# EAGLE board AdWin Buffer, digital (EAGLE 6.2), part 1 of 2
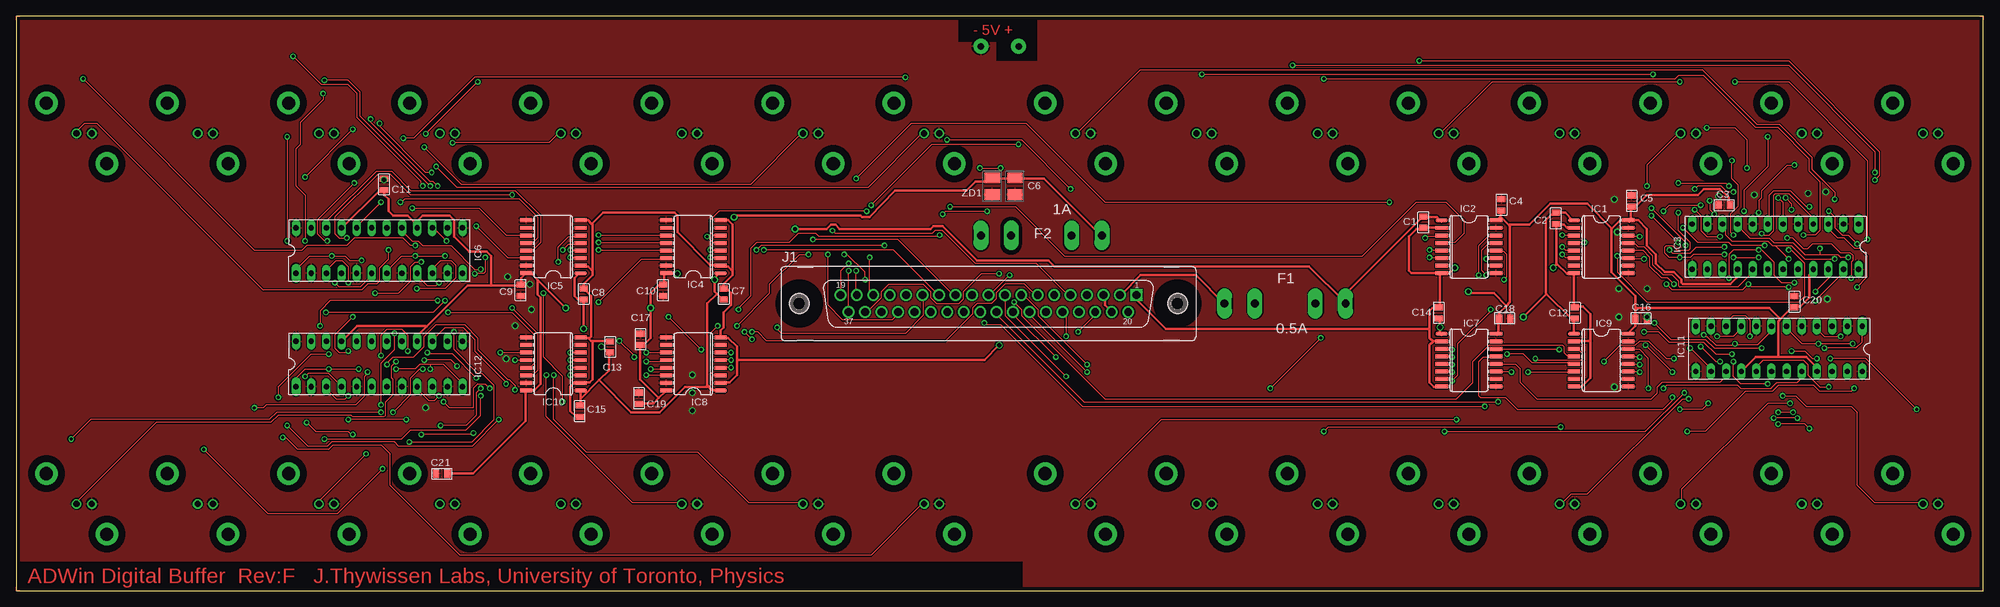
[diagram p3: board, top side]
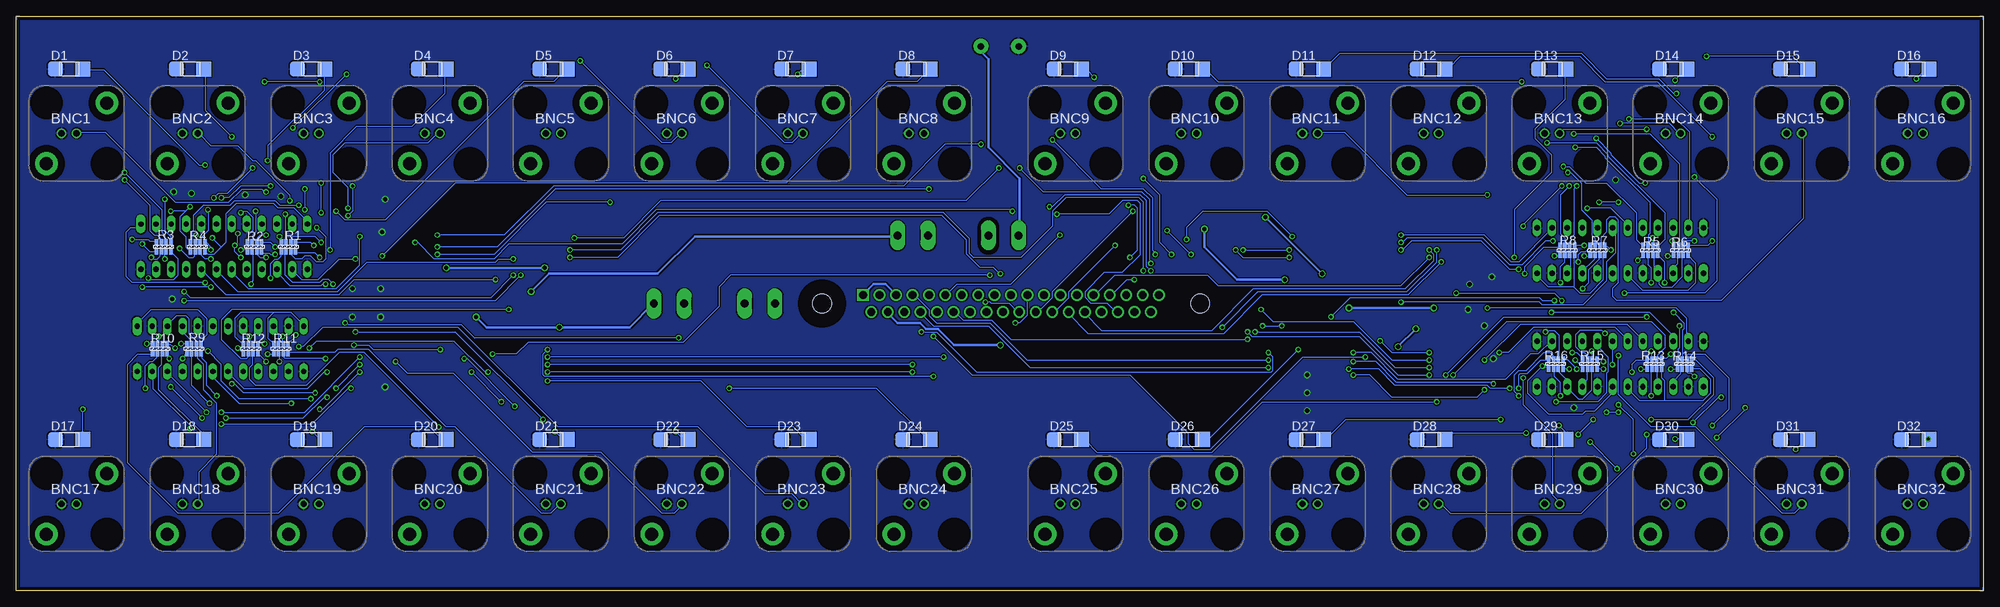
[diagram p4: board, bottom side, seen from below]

Size 330.2 x 96.52 mm. Coordinates in mm from the lower left corner, seen from the top.
Outline: 0,0 330.2,0 330.2,96.52 0,96.52 0,0
Copper layers (1+16): Top 0.035mm / dielectric 1.5mm / Bottom 0.035mm
Design rules: minimum track width 7mil, minimum drill 20mil, track to track 7mil, track to pad 7mil, pad to pad 7mil, via to via 7mil, smd to smd 0mil, copper to edge 25mil, drill to drill 8mil, minimum pad ring 10mil, minimum via ring 8mil, stop-mask expansion 4mil, vias tented up to drill 0mil, thermal gap 10mil
Net classes: 0 default: drill 0.508 mm; 1 PowerA: width 0.406 mm, drill 0.711 mm; 2 Power clearance: width 0.406 mm, drill 0.711 mm, clearance 0.508 mm
tRestrict: area 128.1,45 to 134.7,51.6; area 191.6,45 to 198.2,51.6; 4 lines
bRestrict: area 128.1,45 to 134.7,51.6; area 191.6,45 to 198.2,51.6; 5 lines

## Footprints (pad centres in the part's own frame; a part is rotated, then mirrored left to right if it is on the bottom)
CONN-BNC-AMP-TYPE1VERT = drill 1.067: CONDUCTOR 0,0; SHIELD -2.54,0 | drill 2.184 pad 3.81: MTG1 -5.08,-5.08; MTG2 5.08,5.08
0805 = smd 1.016 x 1.397: 1 -1.905,0; 2 0,0
EIA-B = smd 1.778 x 2.54: 1 -1.4,0; 2 1.4,0
1209 = smd 2.5 x 2.5: A 2.3,0; K -2.3,0
FUSE = drill 1.321 pad 2.54 long: 1A -10.16,0; 1B -5.08,0; 2A 10.16,0; 2B 5.08,0
SOIC-16W = smd 0.66 x 2.032: 1 -6.35,-4.572; 2 -5.08,-4.572; 3 -3.81,-4.572; 4 -2.54,-4.572; 5 -1.27,-4.572; 6 0,-4.572; 7 1.27,-4.572; 8 2.54,-4.572; 9 2.54,4.572; 10 1.27,4.572; 11 0,4.572; 12 -1.27,4.572; 13 -2.54,4.572; 14 -3.81,4.572; 15 -5.08,4.572; 16 -6.35,4.572
DIL24 = drill 0.889 pad 1.575 long: 1 -11.43,-3.81 | drill 0.889 long: 2 -8.89,-3.81; 3 -6.35,-3.81; 4 -3.81,-3.81; 5 -1.27,-3.81; 6 1.27,-3.81; 7 3.81,-3.81; 8 6.35,-3.81; 9 8.89,-3.81; 10 11.43,-3.81; 11 13.97,-3.81; 12 16.51,-3.81; 13 16.51,3.81; 14 13.97,3.81; 15 11.43,3.81; 16 8.89,3.81; 17 6.35,3.81; 18 3.81,3.81; 19 1.27,3.81; 20 -1.27,3.81; 21 -3.81,3.81; 22 -6.35,3.81; 23 -8.89,3.81; 24 -11.43,3.81
CONN:DB37-VERT = drill 1.321 square: 1 24.841,1.422 | drill 1.321: 2 22.073,1.422; 3 19.329,1.422; 4 16.561,1.422; 5 13.792,1.422; 6 11.049,1.422; 7 8.28,1.422; 8 5.512,1.422; 9 2.769,1.422; 10 0,1.422; 11 -2.769,1.422; 12 -5.512,1.422; 13 -8.28,1.422; 14 -11.049,1.422; 15 -13.818,1.422; 16 -16.561,1.422; 17 -19.329,1.422; 18 -22.098,1.422; 19 -24.841,1.422; 20 23.47,-1.422; 21 20.701,-1.422; 22 17.932,-1.422; 23 15.189,-1.422; 24 12.421,-1.422; 25 9.652,-1.422; 26 6.909,-1.422; 27 4.14,-1.422; 28 1.372,-1.422; 29 -1.372,-1.422; 30 -4.14,-1.422; 31 -6.909,-1.422; 32 -9.677,-1.422; 33 -12.421,-1.422; 34 -15.189,-1.422; 35 -17.958,-1.422; 36 -20.701,-1.422; 37 -23.47,-1.422 | hole 3.175: 31.75,0; -31.75,0
PANASONIC_EXB-V8V(QUAD-R-PACK) = smd 1 x 0.59: 1A -0.8,1.2; 1B 0.8,1.2; 2A -0.8,0.4; 2B 0.8,0.4; 3A -0.8,-0.4; 3B 0.8,-0.4; 4A -0.8,-1.2; 4B 0.8,-1.2
TP-HOLE = drill 1.067 pad 2.54: P$1 0,0

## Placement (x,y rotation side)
BNC1  AMP 227673-1  [CONN-BNC-AMP-TYPE1VERT]  320.04,76.83 0 bottom
BNC2  AMP 227673-1  [CONN-BNC-AMP-TYPE1VERT]  299.72,76.83 0 bottom
BNC3  AMP 227673-1  [CONN-BNC-AMP-TYPE1VERT]  279.4,76.83 0 bottom
BNC4  AMP 227673-1  [CONN-BNC-AMP-TYPE1VERT]  259.08,76.83 0 bottom
BNC5  AMP 227673-1  [CONN-BNC-AMP-TYPE1VERT]  238.76,76.83 0 bottom
BNC6  AMP 227673-1  [CONN-BNC-AMP-TYPE1VERT]  218.44,76.83 0 bottom
BNC7  AMP 227673-1  [CONN-BNC-AMP-TYPE1VERT]  198.12,76.83 0 bottom
BNC8  AMP 227673-1  [CONN-BNC-AMP-TYPE1VERT]  177.8,76.83 0 bottom
BNC9  AMP 227673-1  [CONN-BNC-AMP-TYPE1VERT]  152.4,76.83 0 bottom
BNC10  AMP 227673-1  [CONN-BNC-AMP-TYPE1VERT]  132.08,76.83 0 bottom
BNC11  AMP 227673-1  [CONN-BNC-AMP-TYPE1VERT]  111.76,76.83 0 bottom
BNC12  AMP 227673-1  [CONN-BNC-AMP-TYPE1VERT]  91.44,76.83 0 bottom
BNC13  AMP 227673-1  [CONN-BNC-AMP-TYPE1VERT]  71.12,76.83 0 bottom
BNC14  AMP 227673-1  [CONN-BNC-AMP-TYPE1VERT]  50.8,76.83 0 bottom
BNC15  AMP 227673-1  [CONN-BNC-AMP-TYPE1VERT]  30.48,76.83 0 bottom
BNC16  AMP 227673-1  [CONN-BNC-AMP-TYPE1VERT]  10.16,76.83 0 bottom
BNC17  AMP 227673-1  [CONN-BNC-AMP-TYPE1VERT]  320.04,14.61 0 bottom
BNC18  AMP 227673-1  [CONN-BNC-AMP-TYPE1VERT]  299.72,14.61 0 bottom
BNC19  AMP 227673-1  [CONN-BNC-AMP-TYPE1VERT]  279.4,14.61 0 bottom
BNC20  AMP 227673-1  [CONN-BNC-AMP-TYPE1VERT]  259.08,14.61 0 bottom
BNC21  AMP 227673-1  [CONN-BNC-AMP-TYPE1VERT]  238.76,14.61 0 bottom
BNC22  AMP 227673-1  [CONN-BNC-AMP-TYPE1VERT]  218.44,14.61 0 bottom
BNC23  AMP 227673-1  [CONN-BNC-AMP-TYPE1VERT]  198.12,14.61 0 bottom
BNC24  AMP 227673-1  [CONN-BNC-AMP-TYPE1VERT]  177.8,14.61 0 bottom
BNC25  AMP 227673-1  [CONN-BNC-AMP-TYPE1VERT]  152.4,14.61 0 bottom
BNC26  AMP 227673-1  [CONN-BNC-AMP-TYPE1VERT]  132.08,14.61 0 bottom
BNC27  AMP 227673-1  [CONN-BNC-AMP-TYPE1VERT]  111.76,14.61 0 bottom
BNC28  AMP 227673-1  [CONN-BNC-AMP-TYPE1VERT]  91.44,14.61 0 bottom
BNC29  AMP 227673-1  [CONN-BNC-AMP-TYPE1VERT]  71.12,14.61 0 bottom
BNC30  AMP 227673-1  [CONN-BNC-AMP-TYPE1VERT]  50.8,14.61 0 bottom
BNC31  AMP 227673-1  [CONN-BNC-AMP-TYPE1VERT]  30.48,14.61 0 bottom
BNC32  AMP 227673-1  [CONN-BNC-AMP-TYPE1VERT]  10.16,14.61 0 bottom
C1  0.1uF  [0805]  236.22,62.87 90 top
C2  0.1uF  [0805]  258.44,63.5 90 top
C3  0.1uF  [0805]  287.65,64.77 0 top
C4  0.1uF  [0805]  249.3,63.88 270 top
C5  0.1uF  [0805]  271.14,64.52 270 top
C6  4.7uF  [EIA-B]  167.64,67.94 90 top
C7  0.1uF  [0805]  118.75,48.9 270 top
C8  0.1uF  [0805]  95.25,48.9 270 top
C9  0.1uF  [0805]  84.71,51.44 90 top
C10  0.1uF  [0805]  108.58,51.44 90 top
C11  0.1uF  [0805]  61.72,67.31 270 top
C12  0.1uF  [0805]  261.62,45.72 270 top
C13  0.1uF  [0805]  99.69,40.01 270 top
C14  0.1uF  [0805]  238.76,45.72 270 top
C15  0.1uF  [0805]  94.61,31.11 90 top
C16  0.1uF  [0805]  271.78,45.72 180 top
C17  0.1uF  [0805]  104.78,41.27 270 top
C18  0.1uF  [0805]  248.92,45.72 180 top
C19  0.1uF  [0805]  104.52,31.37 270 top
C20  0.1uF  [0805]  298.45,47.62 270 top
C21  0.1uF  [0805]  72.39,19.68 0 top
D1  [1209]  321.31,87.63 0 bottom
D2  [1209]  300.99,87.63 0 bottom
D3  [1209]  280.67,87.63 0 bottom
D4  [1209]  260.35,87.63 0 bottom
D5  [1209]  240.03,87.63 0 bottom
D6  [1209]  219.71,87.63 0 bottom
D7  [1209]  199.39,87.63 0 bottom
D8  [1209]  179.07,87.63 0 bottom
D9  [1209]  153.67,87.63 0 bottom
D10  [1209]  133.35,87.63 0 bottom
D11  [1209]  113.03,87.63 0 bottom
D12  [1209]  92.71,87.63 0 bottom
D13  [1209]  72.39,87.63 0 bottom
D14  [1209]  52.07,87.63 0 bottom
D15  [1209]  31.75,87.63 0 bottom
D16  [1209]  11.43,87.63 0 bottom
D17  [1209]  321.31,25.4 0 bottom
D18  [1209]  300.99,25.4 0 bottom
D19  [1209]  280.67,25.4 0 bottom
D20  [1209]  260.35,25.4 0 bottom
D21  [1209]  240.03,25.4 0 bottom
D22  [1209]  219.71,25.4 0 bottom
D23  [1209]  199.39,25.4 0 bottom
D24  [1209]  179.07,25.4 0 bottom
D25  [1209]  153.67,25.4 0 bottom
D26  [1209]  133.35,25.4 0 bottom
D27  [1209]  113.03,25.4 0 bottom
D28  [1209]  92.71,25.4 0 bottom
D29  [1209]  72.39,25.4 0 bottom
D30  [1209]  52.07,25.4 0 bottom
D31  [1209]  31.75,25.4 0 bottom
D32  [1209]  11.43,25.4 0 bottom
F1  0.5A  [FUSE]  213,48.26 0 top
F2  1A  [FUSE]  172.09,59.69 180 top
IC1  ADUM1400BRW  [SOIC-16W]  266.06,55.88 270 top
IC2  ADUM1400BRW  [SOIC-16W]  243.84,55.88 270 top
IC3  SN64BCT25244NT  [DIL24]  297.83,57.8 180 top
IC4  ADUM1400BRW  [SOIC-16W]  113.67,59.69 90 top
IC5  ADUM1400BRW  [SOIC-16W]  90.17,59.69 90 top
IC6  SN64BCT25244NT  [DIL24]  58.42,57.15 0 top
IC7  ADUM1400BRW  [SOIC-16W]  243.84,36.83 270 top
IC8  ADUM1400BRW  [SOIC-16W]  113.67,40.01 90 top
IC9  ADUM1400BRW  [SOIC-16W]  266.06,36.83 270 top
IC10  ADUM1400BRW  [SOIC-16W]  90.17,40.01 90 top
IC11  SN64BCT25244NT  [DIL24]  298.45,40.64 180 top
IC12  SN64BCT25244NT  [DIL24]  58.42,38.1 0 top
J1  Norcomp 191-037-223R001  [CONN:DB37-VERT]  163.19,48.26 0 top
R1  47  [PANASONIC_EXB-V8V(QUAD-R-PACK)]  284.48,57.78 90 bottom
R2  470  [PANASONIC_EXB-V8V(QUAD-R-PACK)]  290.19,57.78 90 bottom
R3  47  [PANASONIC_EXB-V8V(QUAD-R-PACK)]  305.44,57.78 90 bottom
R4  470  [PANASONIC_EXB-V8V(QUAD-R-PACK)]  299.72,57.78 90 bottom
R5  47  [PANASONIC_EXB-V8V(QUAD-R-PACK)]  55.88,57.15 90 bottom
R6  470  [PANASONIC_EXB-V8V(QUAD-R-PACK)]  50.8,57.15 90 bottom
R7  47  [PANASONIC_EXB-V8V(QUAD-R-PACK)]  64.77,57.15 90 bottom
R8  470  [PANASONIC_EXB-V8V(QUAD-R-PACK)]  69.85,57.15 90 bottom
R9  47  [PANASONIC_EXB-V8V(QUAD-R-PACK)]  300.36,40.64 270 bottom
R10  470  [PANASONIC_EXB-V8V(QUAD-R-PACK)]  306.07,40.64 270 bottom
R11  47  [PANASONIC_EXB-V8V(QUAD-R-PACK)]  285.75,40.64 270 bottom
R12  470  [PANASONIC_EXB-V8V(QUAD-R-PACK)]  290.83,40.64 270 bottom
R13  47  [PANASONIC_EXB-V8V(QUAD-R-PACK)]  55.24,38.1 90 bottom
R14  470  [PANASONIC_EXB-V8V(QUAD-R-PACK)]  50.16,38.1 90 bottom
R15  47  [PANASONIC_EXB-V8V(QUAD-R-PACK)]  66.04,38.1 90 bottom
R16  470  [PANASONIC_EXB-V8V(QUAD-R-PACK)]  71.75,38.1 90 bottom
SUPPLY_+5V  [TP-HOLE]  168.28,91.44 0 top
SUPPLY_RETURN  [TP-HOLE]  161.93,91.44 0 top
U$19  [TITLEBLOCK_PCB]  not placed on the board
ZD1  1N5339  [EIA-B]  163.83,67.94 90 top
